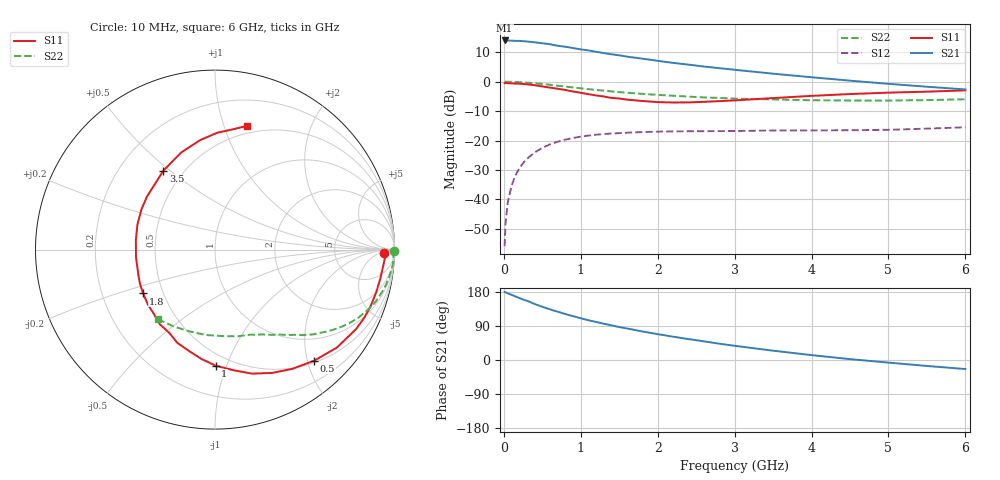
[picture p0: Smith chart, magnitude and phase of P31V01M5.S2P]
! SIEMENS Small Signal Semiconductors
! BFP181
! Si NPN RF Bipolar Junction Transistor in SOT143
! VCE = 1 V  IC = 1.5 mA
! Common Emitter S-Parameters:  March  1996
# GHz  S  MA  R  50
!  f  S11  S21  S12  S22
! GHz  MAG  ANG  MAG  ANG  MAG  ANG  MAG  ANG
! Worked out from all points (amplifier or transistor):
!   36 points, 10 MHz to 6 GHz, reference 50 ohm
!   highest |S21| = 14.0 dB at 10 MHz (marker M1)
!   |S21| within 3 dB of that: start of sweep to 992.9 MHz
!   unconditionally stable (mu >= 1): 2.532 GHz to end of sweep
!   at 250 MHz: K = 0.12, MSG = 20.7 dB, |S12| = -27.7 dB
!   at 1.4 GHz: K = 0.61, MSG = 13.5 dB, |S12| = -17.6 dB
!   at 6 GHz: K = 1.26, MAG = 3.4 dB, |S12| = -15.5 dB
!   S11 on the Smith chart (normalised r, x): 10 MHz: 31, -10; 500 MHz: 0.53, -2.12; 1 GHz: 0.41, -0.92; 1.8 GHz: 0.39, -0.24; 3.5 GHz: 0.39, +0.48; 6 GHz: 0.43, +1.20
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0.01  0.9436 -1.1  5.015 179.5  0.0016 85.8  0.9973 -0.4
0.02  0.9497 -2.1  5.001 179.0  0.0036 85.3  0.9958 -1.0
0.05  0.9433 -4.7  5.008 176.0  0.0087 89.5  0.9947 -2.4
0.1  0.9351 -10.1  4.974 171.9  0.017 81.8  0.9941 -4.7
0.15  0.929 -14.9  4.936 167.8  0.0254 80.1  0.9877 -7.1
0.25  0.914 -24.6  4.876 159.6  0.0412 74.3  0.9724 -11.7
0.3  0.9022 -29.4  4.816 156.3  0.0487 71.3  0.9625 -13.8
0.4  0.8712 -38.8  4.667 147.9  0.0625 65.8  0.9409 -18.0
0.5  0.8298 -48.2  4.493 140.4  0.0749 60.4  0.9129 -21.8
0.6  0.792 -57.0  4.33 133.7  0.0863 55.3  0.8839 -25.5
0.8  0.7215 -73.3  3.921 121.3  0.1035 46.7  0.8253 -31.4
1  0.6466 -89.7  3.537 110.2  0.1163 39.5  0.7714 -36.3
1.1  0.6133 -97.2  3.396 104.9  0.1212 36.6  0.746 -38.5
1.3  0.5602 -112.0  3.063 95.7  0.1287 30.7  0.7029 -42.4
1.5  0.5171 -126.5  2.803 87.0  0.1333 26.4  0.6638 -45.6
1.8  0.4691 -148.6  2.459 75.3  0.1389 21.5  0.6208 -49.8
2.2  0.4422 -174.5  2.085 61.5  0.1428 15.7  0.5763 -55.5
2.8  0.4666 151.6  1.696 43.1  0.1445 10.6  0.5289 -64.0
3.5  0.5259 123.1  1.366 24.6  0.1479 6.6  0.4991 -75.4
4.5  0.6156 97.7  1.04 2.3  0.1495 3.2  0.4784 -95.9
5.5  0.6758 81.9  0.82 -15.7  0.1592 3.2  0.4862 -118.2
6  0.711 75.6  0.738 -23.8  0.1677 2.1  0.5013 -129.4
